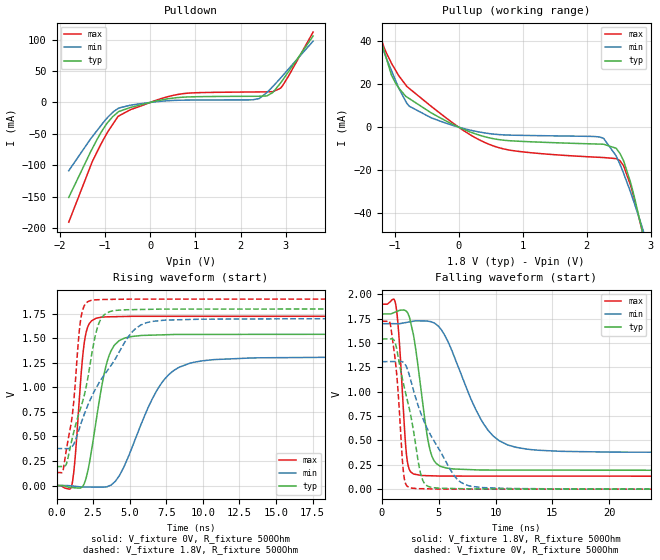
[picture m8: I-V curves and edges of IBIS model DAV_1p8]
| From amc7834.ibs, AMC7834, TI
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|   Model
[Model]   DAV_1p8
Model_type   Output
Polarity   Non-Inverting
Vmeas = 0.9
Vref = 0
Cref = 1pF
Rref = 100000
|   typ   min   max
C_comp   3.504pF   3.144pF   3.899pF
[Voltage Range]   1.8   1.7   1.9
[Temperature Range]   27   125   -40
[Pullup Reference]   1.8   1.7   1.9
[Pulldown Reference]   0   0   0
[Power Clamp Reference]   1.8   1.7   1.9
[GND Clamp Reference]   0   0   0
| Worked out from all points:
|   slope of the pulldown table from 0 to 0.27 V, typ, clamps not added: 62.8 ohm
|   slope of the pullup table from 0 to 0.27 V, typ, clamps not added: 84 ohm
|   falling waveform, V_fixture 1.8V, R_fixture 500Ohm: 20-80 % time 1.11ns typ, 3.01ns min, 552ps max; typ from 1.8 V to 0.193 V
|   rising waveform, V_fixture 0V, R_fixture 500Ohm: 20-80 % time 1.07ns typ, 2.38ns min, 528ps max; typ from 0 V to 1.54 V
|   rising waveform, V_fixture 1.8V, R_fixture 500Ohm: 20-80 % time 1.45ns typ, 2.87ns min, 720ps max; typ from 0.193 V to 1.8 V
|   falling waveform, V_fixture 0V, R_fixture 500Ohm: 20-80 % time 1.53ns typ, 3.03ns min, 660ps max; typ from 1.54 V to 0 V
[Pulldown]
|   Voltage   I(typ)   I(min)   I(max)
-1.8V     -151mA     -108.6mA   -190.5mA
-1.275V   -72.75mA   -54.02mA   -93.18mA
-979.3mV  -35.71mA   -26.92mA   -52.01mA
-709.2mV  -15.24mA   -9.654mA   -22.03mA
111.6mV   1.936mA    948.2uA    2.988mA
689.4mV   8.196mA    3.58mA     13.6mA
2.266V    9.809mA    4.163mA    16.64mA
2.412V    9.853mA    6.303mA    16.72mA
2.579V    10.37mA    15.75mA    16.81mA
2.714V    16.21mA    25.67mA    17.2mA
2.925V    35.27mA    42.3mA     26.64mA
3.6V      105.7mA    97.5mA     111.9mA
[Pullup]
|   Voltage   I(typ)   I(min)   I(max)
-1.8V     98.11mA    86.45mA    111.9mA
-1.275V   46.43mA    43.92mA    47.66mA
-1.049V   24.22mA    26.39mA    29.79mA
-774mV    13.37mA    9.804mA    18.09mA
-61.2mV   859.7uA    538.4uA    1.32mA
538.2mV   -5.36mA    -3.219mA   -8.715mA
2.25V     -7.965mA   -5.034mA   -14.16mA
2.461V    -9.845mA   -13.37mA   -14.68mA
2.574V    -15.48mA   -21.23mA   -17.84mA
2.687V    -25.87mA   -30.41mA   -27.19mA
2.866V    -47.97mA   -46.48mA   -48.1mA
3.6V      -156.5mA   -123.2mA   -179.6mA
[Ramp]
R_load = 500
|   typ   min   max
dV/dt_r   0.925714/1.06844e-09   0.785788/2.3821e-09   1.0351/5.28179e-10
dV/dt_f   0.963998/1.11351e-09   0.793253/2.99672e-09   1.06009/5.51965e-10
[Falling Waveform]
V_fixture = 1.8V
V_fixture_min = 1.7V
V_fixture_max = 1.9V
R_fixture = 500Ohm
C_fixture = 0F
|   Time   V(typ)   V(min)   V(max)
0s        1.8V       1.7V       1.9V
1.248ns   1.822V     1.7V       1.879V
1.539ns   1.836V     1.7V       1.513V
2.164ns   1.828V     1.713V     359.1mV
2.752ns   1.6V       1.725V     158.7mV
4.155ns   444.7mV    1.723V     138mV
5.134ns   235.6mV    1.652V     134.5mV
8.692ns   196.7mV    721.2mV    134.3mV
11.04ns   196.3mV    456.2mV    134.2mV
30ns      193.3mV    377.9mV    133.2mV
[Rising Waveform]
V_fixture = 0V
V_fixture_min = 0V
V_fixture_max = 0V
R_fixture = 500Ohm
C_fixture = 0F
|   Time   V(typ)   V(min)   V(max)
0s        1.525uV    -4.688uV   59.61nV
1.082ns   -21.02mV   -4.965mV   29.1mV
1.91ns    25.72mV    -15.17mV   1.469V
2.202ns   195.3mV    -15.53mV   1.64V
2.661ns   616.2mV    -16.09mV   1.702V
3.386ns   1.224V     -13.81mV   1.719V
3.983ns   1.435V     38.19mV    1.721V
7.022ns   1.535V     1.01V      1.724V
9.04ns    1.539V     1.243V     1.724V
30ns      1.543V     1.31V      1.725V
[Rising Waveform]
V_fixture = 1.8V
V_fixture_min = 1.7V
V_fixture_max = 1.9V
R_fixture = 500Ohm
C_fixture = 0F
|   Time   V(typ)   V(min)   V(max)
0s        193.3mV    377.7mV    133.2mV
461.3ps   194.1mV    376.6mV    163.6mV
1.082ns   485.4mV    400mV      720mV
1.66ns    796.6mV    626.3mV    1.701V
2.25ns    1.195V     856.9mV    1.881V
2.631ns   1.517V     974.6mV    1.892V
3.162ns   1.725V     1.106V     1.896V
5.212ns   1.792V     1.572V     1.899V
6.35ns    1.795V     1.667V     1.899V
30ns      1.8V       1.7V       1.9V
[Falling Waveform]
|Gnd
V_fixture = 0V
V_fixture_min = 0V
V_fixture_max = 0V
R_fixture = 500Ohm
C_fixture = 0F
|   Time   V(typ)   V(min)   V(max)
0s        1.543V     1.31V      1.725V
781.9ps   1.544V     1.311V     1.672V
1.343ns   1.418V     1.312V     1.131V
1.91ns    1.079V     1.301V     165.7mV
2.356ns   856.8mV    1.195V     19.81mV
3.302ns   217.6mV    821.7mV    5.315mV
3.707ns   66.63mV    697.3mV    4.348mV
6.35ns    6.557mV    140.5mV    941.8uV
7.425ns   3.668mV    43.16mV    899.1uV
30ns      -6.491uV   68.12uV    901.6nV
